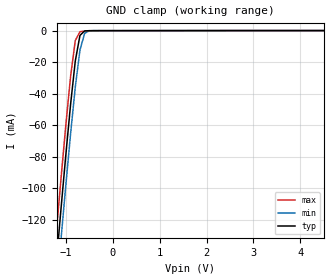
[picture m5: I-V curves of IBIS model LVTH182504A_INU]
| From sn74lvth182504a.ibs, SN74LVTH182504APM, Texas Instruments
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[Model]   LVTH182504A_INU
| input buffer with pullup resistor
| inup.lvta (97212 ALEY)
| pad.lvta  (97212 ALEY)
| Signals   OE#, TDI, TMS
Model_type  Input
Polarity   Non-Inverting
Vinl = 0.8V
Vinh = 2.0V
| variable   typ   min   max
C_comp   4p   NA   NA
[Temperature Range]   50   100   0
[Voltage range]   3.3   3   3.6
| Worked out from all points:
|   GND clamp passes 1 mA (typ) near -0.63 V on its own axis
|Process range|   weak   strong
[gnd_clamp]
|   50C:3.3V:   100C:3V:weak   0C:3.6V:strong
|   Voltage   I(typ)   I(min)   I(max)
-3.3V     -902.8mA   -920.5mA   -885.5mA
-1.2V     -145.7mA   -165.1mA   -126.6mA
-1.1V     -111.6mA   -131mA     -92.5mA
-1V       -78.36mA   -97.59mA   -59.5mA
-900mV    -46.85mA   -65.49mA   -29.04mA
-800mV    -19.34mA   -35.91mA   -6.369mA
-700mV    -3.045mA   -12.31mA   -672.7uA
-600mV    -219.4uA   -1.707mA   -305.5uA
-500mV    -55.08uA   -153.2uA   -130.6uA
6.6V      2.311nA    2.461nA    2.28nA
